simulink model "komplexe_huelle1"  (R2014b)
settings: Solver=ode45  StartTime=0.0  StopTime=10.0  RelTol=1e-3
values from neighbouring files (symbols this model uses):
  fs = 1000    [abtast_fir_1.m]    (also in abtast_fir_2.m; abtast_fir_3.m; abtast_fir_4.m; hilbert_filter_1.m)
  hd = Hd.numerator    [fdesign_1.m]    (also in grp_komp_1.m = fdesign.lowpass('N,Fp,Ap,Ast',nord,fr,dp,ds); hilbert_filter_1.m = design(d, 'equiripple'); hilbert_filter_2.m = design(d, 'equiripple'); hilbert_filter_3.m = design(d, 'equiripple'))
  Ts = 1/fs    (= 0.001)    [abtast_fir_1.m]    (also in abtast_fir_2.m; abtast_fir_3.m; abtast_fir_4.m; hilbert_filter_1.m)
undefined symbols (not defined in the file or in its folder): fir1, Fs, get
libraries: dspstat3 x3, dsparch4 x1, dspspect3 x1, dspsnks4 x1

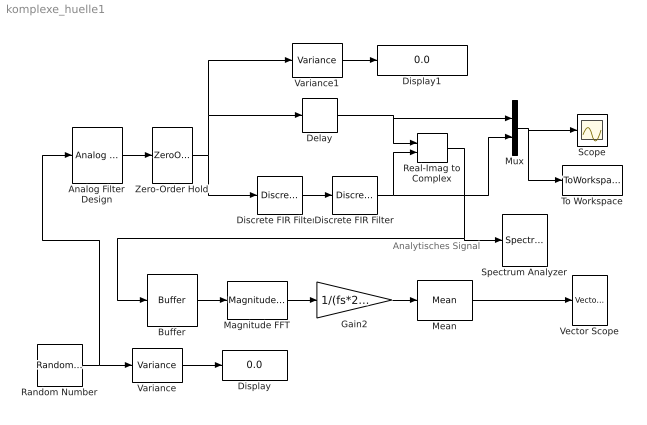
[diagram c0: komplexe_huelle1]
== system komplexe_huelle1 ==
  note: Analytisches Signal
  Analog Filter Design : dsparch4/Analog Filter Design  method=Elliptic  filttype=Bandpass  N=8  Wlo=2*pi*20  Whi=2*pi*400  Rp=2  Rs=40
  Buffer : Buffer  N=256  TreatMby1Signals=One channel
  Delay : Delay  DelayLength=96  UseCircularBuffer=on  SampleTime=Ts
  Discrete FIR Filter : DiscreteFir  Coefficients=hd.numerator
  Discrete FIR Filter1 : DiscreteFir  Coefficients=fir1(128, 0.3)  SampleTime=Ts
  Display : Display
  Display1 : Display
  Gain2 : Gain  Gain=1/(fs*256)
  Magnitude FFT : dspspect3/Magnitude FFT  mag_or_magsq=Magnitude squared  FFTImplementation=Auto  fftLenInherit=on  fftsize=256  WrapInput=off
  Mean : dspstat3/Mean  run=on  reset_popup=None  directionMode=Each column  dimension=1  treatSBRowAsCol=on  roiEnable=off  roiType=Rectangles  roiPortion=Entire ROI  roiOutput=Individual statistics for each ROI  roiFlag=off  outputDataTypeStr=Inherit: Same as accumulator  outputLastDataTypeStr=Inherit: Same as accumulator  outputMin=[]  outputMax=[]  roundingMode=Floor  overflowMode=off
  Mux : Mux  Inputs=2
  Random Number : RandomNumber  SampleTime=Ts/10
  Real-Imag to Complex : RealImagToComplex
  Scope : Scope
  Spectrum Analyzer : SpectrumAnalyzer
  To Workspace : ToWorkspace  VariableName=y  SaveFormat=Timeseries  SampleTime=-1
  Variance : dspstat3/Variance  run=on  reset_popup=None  InputProcessing=Columns as channels (frame based)  directionMode=Each column  dimension=1  treatSBRowAsCol=on  roiEnable=off  roiType=Rectangles  roiPortion=Entire ROI  roiOutput=Individual statistics for each ROI  roiFlag=off  roundingMode=Floor  overflowMode=off
  Variance1 : dspstat3/Variance  run=on  reset_popup=None  InputProcessing=Columns as channels (frame based)  directionMode=Each column  dimension=1  treatSBRowAsCol=on  roiEnable=off  roiType=Rectangles  roiPortion=Entire ROI  roiOutput=Individual statistics for each ROI  roiFlag=off  roundingMode=Floor  overflowMode=off
  Vector Scope : dspsnks4/Vector Scope  ScopeProperties=on  Domain=Frequency  HorizSpan=1  DisplayProperties=off  AxisGrid=on  Memory=off  FrameNumber=on  AxisLegend=off  AxisZoom=off  OpenScopeAtSimStart=on  OpenScopeImmediately=off  FigPos=get(0,'defaultfigureposition')  AxisProperties=off  XUnits=Hertz  XRange=[-Fs/2...Fs/2]  InheritXIncr=off  XIncr=Ts  XLabel=Time  XLimit=User-defined  XMin=-500  XMax=500  XStart=0  YUnits=dB  YLabel=Amplitude  LineProperties=off  XAxisParamsVer=6.9
  Zero-Order Hold : ZeroOrderHold  SampleTime=Ts
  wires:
  Analog Filter Design/1 -> Zero-Order Hold/1
  Mux/1 -> To Workspace/1, Scope/1
  Discrete FIR Filter/1 -> Real-Imag to Complex/2, Mux/2
  Delay/1 -> Mux/1, Real-Imag to Complex/1
  Variance/1 -> Display/1
  Variance1/1 -> Display1/1
  Random Number/1 -> Analog Filter Design/1, Variance/1
  Real-Imag to Complex/1 -> Buffer/1, Spectrum Analyzer/1
  Zero-Order Hold/1 -> Discrete FIR Filter1/1, Delay/1, Variance1/1
  Magnitude FFT/1 -> Gain2/1
  Gain2/1 -> Mean/1
  Mean/1 -> Vector Scope/1
  Buffer/1 -> Magnitude FFT/1
  Discrete FIR Filter1/1 -> Discrete FIR Filter/1
